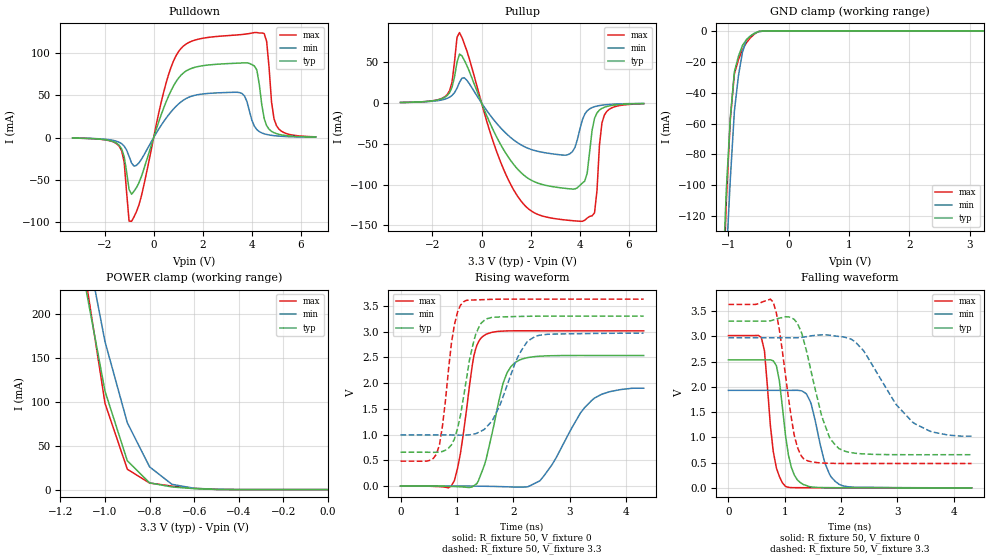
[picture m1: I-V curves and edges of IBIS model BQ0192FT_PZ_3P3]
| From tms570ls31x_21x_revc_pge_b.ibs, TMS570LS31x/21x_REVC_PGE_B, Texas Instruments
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|IQ0442FT_40P60P_PD_3P3; PULLDOWN_ON
|   Model Cell BQ0192FT_PZ_3P3
|BQ0192FT_PZ_3P3
[Model]   BQ0192FT_PZ_3P3
Model_type   I/O
Polarity   Non-Inverting
Enable   Active-Low
Vinl =  1.15
Vinh =  1.55
Cref =  15.0001pF
Rref =  101.0000M
Vref =  0V
Vmeas =  1.65
C_comp   1.2p   1.2p   1.2p
[Model Spec]
Vinl   1.15   1.02   1.28
Vinh   1.55   1.45   1.65
[Temperature Range]   25   155   -40
[Voltage Range]   3.3   2.97   3.63
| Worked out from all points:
|   slope of the pulldown table from 0 to 0.495 V, typ, clamps not added: 11.9 ohm
|   slope of the pullup table from 0 to 0.495 V, typ, clamps not added: 14.3 ohm
|   GND clamp passes 1 mA (typ) near -0.53 V on its own axis
|   POWER clamp passes 1 mA (typ) near -0.59 V on its own axis
|   rising waveform, R_fixture 50, V_fixture 0: 20-80 % time 315ps typ, 599ps min, 226ps max; typ from 0 V to 2.53 V
|   rising waveform, R_fixture 50, V_fixture 3.3: 20-80 % time 266ps typ, 431ps min, 200ps max; typ from 0.657 V to 3.3 V
|   falling waveform, R_fixture 50, V_fixture 0: 20-80 % time 182ps typ, 257ps min, 153ps max; typ from 2.53 V to 0 V
|   falling waveform, R_fixture 50, V_fixture 3.3: 20-80 % time 362ps typ, 700ps min, 237ps max; typ from 3.3 V to 0.657 V
[POWER_clamp]
|   voltage   I(typ)   I(min)   I(max)
-3.3V     4.054A     4.63A      4.887A
-1.1V     248.3mA    301mA      262.7mA
-1.067V   202.9mA    256.9mA    207.9mA
-1.033V   157.5mA    212.7mA    153.1mA
-1V       112.1mA    168.6mA    98.29mA
-900mV    32.88mA    76.23mA    23.22mA
-800mV    7.706mA    25.95mA    7.477mA
-700mV    3.034mA    6.039mA    3.991mA
-600mV    1.088mA    1.528mA    1.425mA
-500mV    187.1uA    369uA      203.4uA
0V        443pA      6.159nA    417pA
[Pulldown]
|   voltage   I(typ)   I(min)   I(max)
-3.3V     -593uA     -522.6uA   -580.3uA
-1.4V     -9.188mA   -5.565mA   -10.35mA
-1.2V     -22.55mA   -10.08mA   -29.13mA
-1V       -61.66mA   -22.23mA   -99.07mA
-900mV    -67.21mA   -30.1mA    -99.29mA
1V        70.16mA    39.61mA    101.5mA
3.5V      88.44mA    53.41mA    122.1mA
4.2V      80.27mA    9.542mA    124.6mA
4.6V      14.18mA    3.749mA    114.2mA
4.8V      7.418mA    2.695mA    42.04mA
5V        4.687mA    2.03mA     14.29mA
6.6V      680.4uA    493.7uA    947.4uA
[Pullup]
|   voltage   I(typ)   I(min)   I(max)
-3.3V     671.9uA    618.2uA    613.1uA
-1.4V     9.171mA    5.687mA    10.35mA
-900mV    59.98mA    25.21mA    86.36mA
600mV     -40.93mA   -24.46mA   -58.45mA
1.4V      -78.76mA   -47.34mA   -111.2mA
3.5V      -105mA     -63.56mA   -143.7mA
4.1V      -98.17mA   -21.1mA    -145.1mA
4.3V      -85.91mA   -9.61mA    -141.1mA
4.6V      -18.69mA   -4.516mA   -134.6mA
4.8V      -8.691mA   -3.128mA   -51.49mA
5V        -5.242mA   -2.297mA   -14.81mA
6.6V      -711.8uA   -541.3uA   -921.2uA
[GND_clamp]
|   voltage   I(typ)   I(min)   I(max)
-3.3V     -3.25A     -2.875A    -4.945A
-1.1V     -166.9mA   -205mA     -187mA
-1.033V   -102.7mA   -146.7mA   -110.1mA
-966.7mV  -55.96mA   -95.69mA   -57.02mA
-900mV    -26.55mA   -52.03mA   -27.8mA
-833.3mV  -16.49mA   -29.28mA   -18.77mA
-766.7mV  -9.539mA   -13.91mA   -12.07mA
-700mV    -5.69mA    -5.924mA   -7.706mA
-566.7mV  -1.567mA   -1.63mA    -2.054mA
-500mV    -402.3uA   -594.3uA   -459.7uA
-366.7mV  -18.7uA    -59.25uA   -17.4uA
3.233V    423.5pA    4.09uA     323pA
[Ramp]
| variable   typ   min   max
dV/dt_f   1.63828/0.3729142n   1.223296/0.7340082n   1.953634/0.2448471n
dV/dt_r   1.540179/0.3172851n   1.17222/0.6246521n   1.831659/0.226962n
R_load = 50
[Rising Waveform]
R_fixture = 50
V_fixture = 0
V_fixture_min = 0
V_fixture_max = 0
|   time   V(typ)   V(min)   V(max)
0s        -4.537uV   -2.498uV   -6.176uV
956ps     -9.905mV   199uV      104.9mV
1.064ns   -15.37mV   128.8uV    635.8mV
1.304ns   7.302mV    -1.954mV   2.538V
1.492ns   415.7mV    -4.662mV   2.929V
1.82ns    1.996V     -12.79mV   3.009V
2.036ns   2.4V       -21.33mV   3.015V
2.472ns   2.521V     99.9mV     3.014V
3.444ns   2.534V     1.708V     3.014V
4.316ns   2.534V     1.9V       3.014V
[Rising Waveform]
R_fixture = 50
V_fixture = 3.3
V_fixture_min = 2.97
V_fixture_max = 3.63
|   time   V(typ)   V(min)   V(max)
0s        656.6mV    993.3mV    482.5mV
640ps     655.6mV    993.3mV    623.4mV
744ps     670.9mV    993.1mV    1.162V
956ps     911.5mV    990.3mV    3.129V
1.116ns   1.712V     987.9mV    3.576V
1.332ns   2.938V     1.017V     3.614V
1.52ns    3.244V     1.138V     3.622V
2.108ns   3.294V     2.562V     3.63V
2.4ns     3.298V     2.911V     3.63V
4.316ns   3.3V       2.969V     3.63V
[Falling Waveform]
R_fixture = 50
V_fixture = 0
V_fixture_min = 0
V_fixture_max = 0
|   time   V(typ)   V(min)   V(max)
0s        2.534V     1.93V      3.014V
584ps     2.533V     1.93V      2.975V
640ps     2.533V     1.93V      2.709V
852ps     2.415V     1.93V      389.9mV
1.012ns   1.047V     1.93V      29.65mV
1.224ns   156.8mV    1.93V      3.728mV
1.44ns    23.47mV    1.739V     1.969mV
1.712ns   5.248mV    491.5mV    537.4uV
1.964ns   2.809mV    70.17mV    298.1uV
4.316ns   87.92uV    820.7uV    7.686uV
[Falling Waveform]
R_fixture = 50
V_fixture = 3.3
V_fixture_min = 2.97
V_fixture_max = 3.63
|   time   V(typ)   V(min)   V(max)
0s        3.3V       2.97V      3.63V
796ps     3.322V     2.97V      3.675V
904ps     3.358V     2.97V      3.127V
1.168ns   3.334V     2.97V      1.04V
1.332ns   2.932V     2.983V     578.7mV
1.656ns   1.417V     3.027V     493.3mV
1.964ns   775.3mV    2.996V     483mV
2.4ns     671.5mV    2.712V     482.4mV
3.268ns   655.7mV    1.301V     482.5mV
4.316ns   656.5mV    1.023V     482.4mV
